(* Logix 5000 AddOnInstructionDefinition export Banner_T30RKU_Param_v4; software revision 33.00 *)

TYPE Banner_IOL_Port_v4 :   // UDT that has all of the data items necessary to communicate with a specific Port on a IO-Link Master
STRUCT
   Port_Controlled : INT;   // Each bit represents a port on an IO-Link Master. Set to 1 to tell AOI to control that port.
   Port_Activate : INT;   // Each bit represents a port on an IO-Link Master. When ON that port will process any commands in queue.
   Port_Read : INT;   // Each bit represents a port on an IO-Link Master. Used to determine when device AOI has requested a Read command.
   Port_Write : INT;   // Each bit represents a port on an IO-Link Master. Used to determine when device AOI has requested a Write command.
   Port_RW_Complete : INT;   // Each bit represents a port on an IO-Link Master. Tells device AOI that Read or Write request has been completed.
   Port_Device_Read : INT;
   Data_Transfer : SINT[190];   // Array to transfer data from IO-Master to device AOIs.
END_STRUCT
END_TYPE

TYPE Banner_T30RKU_RD_v4 :   // UDT that stores the Read Data for a T30RKU.
STRUCT
   Master_Cycle_Time : INT;
   Min_Cycle_Time : INT;
   M_Sequence_Capability : INT;
   IO_Link_Version_ID : INT;
   Process_Data_Input_Length : INT;
   Process_Data_Output_Length : INT;
   Combined_Vendor_ID : DINT;   // IO-Link Vendor ID
   Vendor_ID1 : INT;
   Vendor_ID2 : INT;
   Combined_Device_ID : DINT;   // IO-Link Device ID
   Device_ID1 : INT;
   Device_ID2 : INT;
   Device_ID3 : INT;
   Serial_Number : STRING;
   Teach_State : SINT;
   SP1_TP1 : SINT;
   SP1_TP2 : SINT;
   SP2_TP1 : SINT;
   SP2_TP2 : SINT;
   Distance_Meaurement : DINT;
   Excess_Gain : DINT;   // Amount of singla measured over the minimum threshold.
   Stability : SINT;
   Fault_Status : SINT;   // 0 = No Fault, 1 = Fault Present
   Analog_Output_Value : DINT;
   Temperature : DINT;
   Last_Taught_Temperature : DINT;   // Internal Temperature the last time device was taught.
   All_Time_Run_Time : DINT;   // Read only counter that tracks the total time sensor has been running since manufacture. Value in Hours.
   MDC_Lower_Limit : DINT;
   MDC_Upper_Limit : DINT;
   MDC_Unit : INT;
   MDC_Scale : SINT;
END_STRUCT
END_TYPE

TYPE Banner_T30RKU_v4 :   // All of the parameters for a T30RKU.
STRUCT
   Initial_Global_Read : BOOL;   // Determines if all of the IO-Link data has been read into the PLC yet
   Command : INT;   // Value placed in here will activate a read or write to a specifc IO-Link Index
   Read_Data : Banner_T30RKU_RD_v4;   // Read Only Data
   Write_Data : Banner_T30RKU_WD_v4;   // Write Data
   Archive : Banner_T30RKU_WD_v4;   // Archive Data
   Reset : BOOL;   // Resets AOI. This will force a complete parameter read of the sensor.
END_STRUCT
END_TYPE

TYPE Banner_T30RKU_WD_v4 :   // UDT that stores the Write Data for a T30RKU.
STRUCT
   System_Command : INT;   // See IODD file for list of commands that can be activated via the System Command interface
   Parameter_Access_Lock : SINT;   // Write access to all parameters is prohibited while value is 1. Only this parameter can be adjusted when value is 1.
   Data_Storage_Lock : SINT;   // Automatic data storage is disabled when this value is equal to 1. Read access is not affected.
   Local_Parameterization_Lock : SINT;   // Parameterization via local control elements on device is disabled.
   Local_User_Interface_Lock : SINT;   // Operation of local user interface is disabled.
   Function_Tag : STRING;
   Location_Tag : STRING;
   Teach_in_Channel : SINT;   // 0 = Default, 1 = BDC1, 192 = AO1
   BDC1_Setpoint_1 : DINT;   // 0 to 15000. SP1 switch point in Switch or Window mode.
   BDC1_Setpoint_2 : DINT;   // 0 to 15000. SP2 switch point in Window mode only.
   BDC1_Switchpoint_Logic : INT;   // 0 = Light Operate, 1 = Dark Operate
   BDC1_Mode : SINT;   // 1 = Switch Mode/Single Mode, 2 = Window Mode
   BDC1_Hysteresis : INT;   // 0 to 15000
   Response_Speed : SINT;   // 0 = Fast, 1 = Medium, 2 = Slow
   Peak_Select_Mode : SINT;   // 0 = Strongest Peak, 1 = First Peak
   Sensor_Lockout : SINT;   // 0 = Unlocked, 1 = Locked
   Output_Polarity : SINT;   // 0 = NPN, 1 = PNP
   Process_Data_Filter_Time : INT;
   Process_Data_Layout : SINT;   // 0 = Digital Measurement Sensor, 1 = Distance and Excess Gain, 2 = Distance and Excess Gain with Binary Data
   Remote_Input_Mode : SINT;   // 0 = Disabled, 1 = Teach
   Amplitude_Threshold : DINT;   // 100 to 5000
   Limit_Filter_Enabled : SINT;   // 0 = Disabled, 1 = Enabled. Rate of change filter for the distance measurement.
   Limit_Filter_Hold_Time : DINT;   // 50 to 60000. Hold time for when distance change exceeds configured window.
   Limit_Filter_Positive_Distance : DINT;   // 0 to 1000. Window size for distance changes going away from sensor (set to 0 to disable)
   Limit_Filter_Negative_Distance : DINT;   // 0 to 1000. Window size for distance changes goin towards sensor (set to 0 to disable)
   BDC1_Delay_Timer_1 : DINT;   // 0 to 60000 ms
   BDC1_Delay_Timer_2 : DINT;   // 0 to 60000 ms
   BDC1_Teach_Offset : DINT;   // -15000 to 15000.
   Resettable_Run_Time : DINT;
   AO1_Setpoint_1 : DINT;   // 300 to 15000.
   AO1_Setpoint_2 : DINT;   // 300 to 15000.
   AO1_Output_Type : INT;   // 0 = 4-20 mA, 128 = 0-10V, 129 = .5-4.5V
   AO1_Slope : SINT;   // 0 = Positive, 1 = Negative
   AO1_Loss_of_Signal : SINT;   // 0 = Hold, 1 = Low, 2 = High
   AO1_Average : SINT;   // 0 = 1, 1 = 2, 2= 4, 3 = 8, 4 = 16, 5 = 32, 6 = 64, 7 = 128, 8 = 256, 9 = 512
   All_Time_Run_Time_Event_Time : DINT;
   Resettable_Run_Time_Event_Time : DINT;
   Active_Sensing_Range_Near : DINT;   // 0 to 16000.
   Active_Sensing_Range_Far : DINT;   // 0 to 16000.
END_STRUCT
END_TYPE

ADD_ON_INSTRUCTION Banner_T30RKU_Param_v4   (* revision 4.1, vendor Banner Engineering *)
// AOI to read and write parameter data to an IO-Link T30R Analog.
VAR_IN_OUT
   T30RKU : Banner_T30RKU_v4; {required}
   Port_Data : Banner_IOL_Port_v4; {required}
END_VAR
VAR_INPUT
   Port : DINT; {required}
END_VAR
VAR
   Local_Control : DINT; {access None}
   Global_Read_Command_Value : INT; {access None}
   Global_Write_Command_Value : INT; {access None}
   Command_Being_Processed : BOOL; {access None}
   Update_Archive : BOOL; {access None}
   Index_Write_Inprocess : DINT; {access None}
   Index_Write_Control : DINT; {access None}
   Inprocess_Index : DINT; {access None}
END_VAR

ROUTINE Logic   (* ladder *)
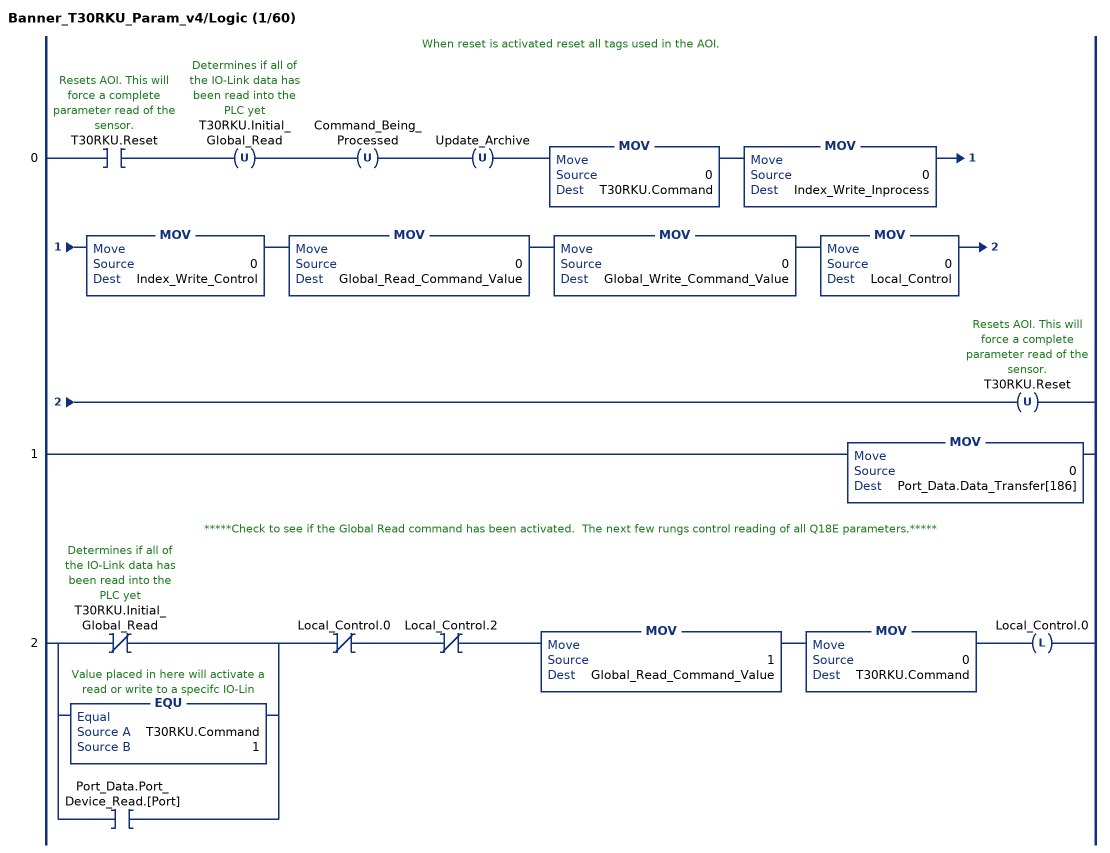
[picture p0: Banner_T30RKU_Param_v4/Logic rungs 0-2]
   // When reset is activated reset all tags used in the AOI.
   0: XIC(T30RKU.Reset)OTU(T30RKU.Initial_Global_Read)OTU(Command_Being_Processed)OTU(Update_Archive)MOV(0,T30RKU.Command)MOV(0,Index_Write_Inprocess)MOV(0,Index_Write_Control)MOV(0,Global_Read_Command_Value)MOV(0,Global_Write_Command_Value)MOV(0,Local_Control)OTU(T30RKU.Reset);
   1: MOV(0,Port_Data.Data_Transfer[186]);
   // *****Check to see if the Global Read command has been activated.  The next few rungs control reading of all Q18E parameters.*****
   2: [XIO(T30RKU.Initial_Global_Read) ,EQU(T30RKU.Command,1) ,XIC(Port_Data.Port_Device_Read.[Port]) ]XIO(Local_Control.0)XIO(Local_Control.2)MOV(1,Global_Read_Command_Value)MOV(0,T30RKU.Command)OTL(Local_Control.0);
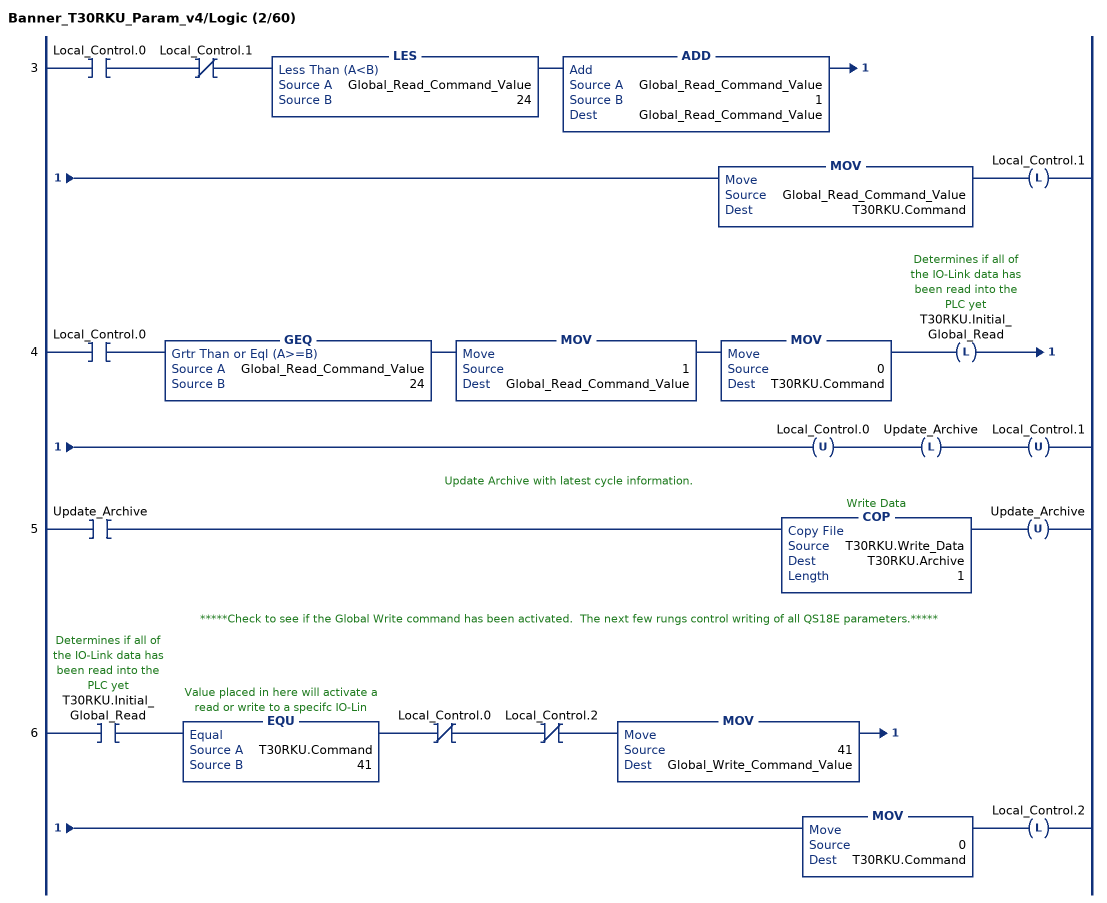
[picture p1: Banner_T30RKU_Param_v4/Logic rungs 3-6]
   3: XIC(Local_Control.0)XIO(Local_Control.1)LES(Global_Read_Command_Value,24)ADD(Global_Read_Command_Value,1,Global_Read_Command_Value)MOV(Global_Read_Command_Value,T30RKU.Command)OTL(Local_Control.1);
   4: XIC(Local_Control.0)GEQ(Global_Read_Command_Value,24)MOV(1,Global_Read_Command_Value)MOV(0,T30RKU.Command)OTL(T30RKU.Initial_Global_Read)OTU(Local_Control.0)OTL(Update_Archive)OTU(Local_Control.1);
   // Update Archive with latest cycle information.
   5: XIC(Update_Archive)COP(T30RKU.Write_Data,T30RKU.Archive,1)OTU(Update_Archive);
   // *****Check to see if the Global Write command has been activated.  The next few rungs control writing of all QS18E parameters.*****
   6: XIC(T30RKU.Initial_Global_Read)EQU(T30RKU.Command,41)XIO(Local_Control.0)XIO(Local_Control.2)MOV(41,Global_Write_Command_Value)MOV(0,T30RKU.Command)OTL(Local_Control.2);
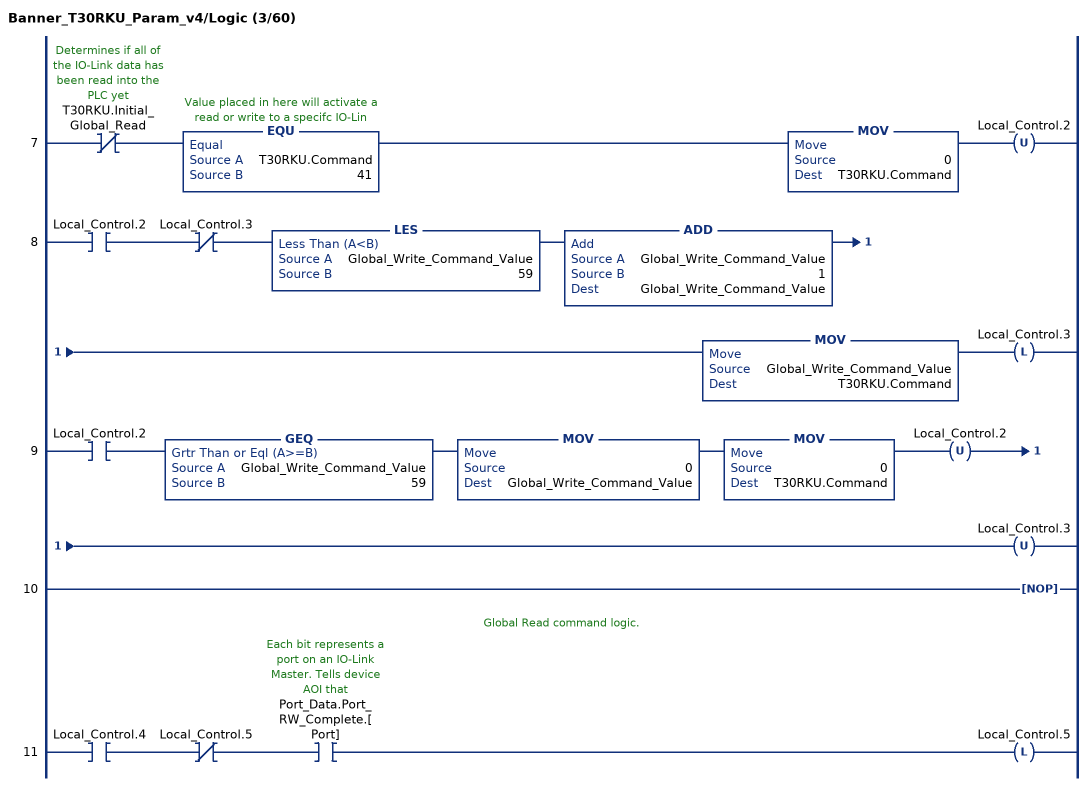
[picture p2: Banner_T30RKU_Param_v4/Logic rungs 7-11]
   7: XIO(T30RKU.Initial_Global_Read)EQU(T30RKU.Command,41)MOV(0,T30RKU.Command)OTU(Local_Control.2);
   8: XIC(Local_Control.2)XIO(Local_Control.3)LES(Global_Write_Command_Value,59)ADD(Global_Write_Command_Value,1,Global_Write_Command_Value)MOV(Global_Write_Command_Value,T30RKU.Command)OTL(Local_Control.3);
   9: XIC(Local_Control.2)GEQ(Global_Write_Command_Value,59)MOV(0,Global_Write_Command_Value)MOV(0,T30RKU.Command)OTU(Local_Control.2)OTU(Local_Control.3);
   10: NOP();
   // Global Read command logic.
   11: XIC(Local_Control.4)XIO(Local_Control.5)XIC(Port_Data.Port_RW_Complete.[Port])OTL(Local_Control.5);
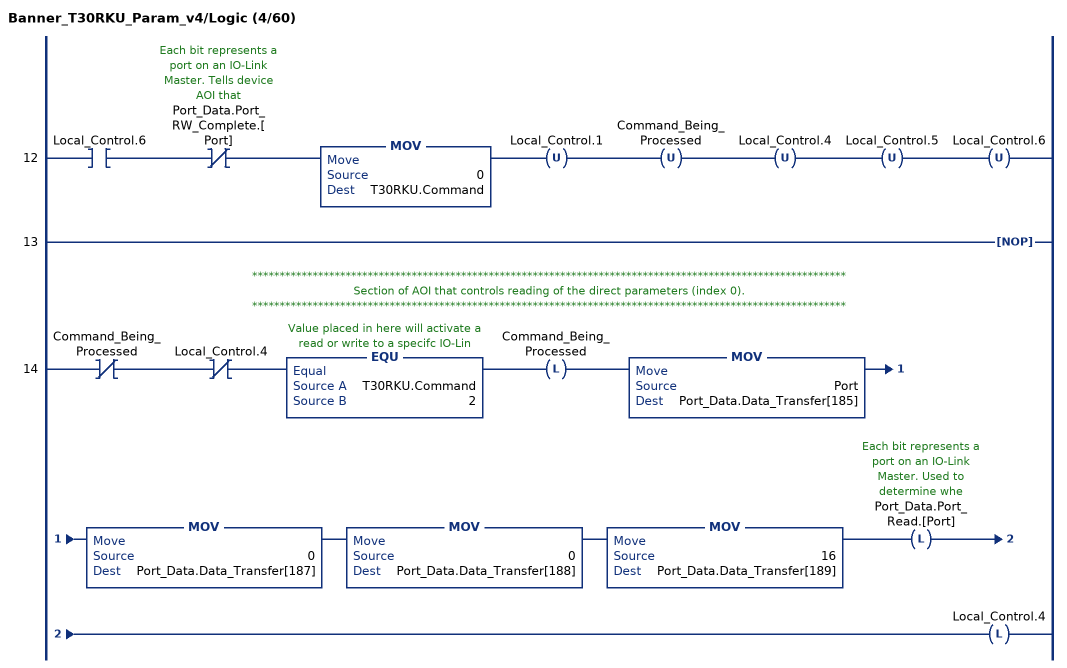
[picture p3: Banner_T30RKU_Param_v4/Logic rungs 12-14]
   12: XIC(Local_Control.6)XIO(Port_Data.Port_RW_Complete.[Port])MOV(0,T30RKU.Command)OTU(Local_Control.1)OTU(Command_Being_Processed)OTU(Local_Control.4)OTU(Local_Control.5)OTU(Local_Control.6);
   13: NOP();
   // ************************************************************************************************************
   // Section of AOI that controls reading of the direct parameters (index 0).
   // ************************************************************************************************************
   14: XIO(Command_Being_Processed)XIO(Local_Control.4)EQU(T30RKU.Command,2)OTL(Command_Being_Processed)MOV(Port,Port_Data.Data_Transfer[185])MOV(0,Port_Data.Data_Transfer[187])MOV(0,Port_Data.Data_Transfer[188])MOV(16,Port_Data.Data_Transfer[189])OTL(Port_Data.Port_Read.[Port])OTL(Local_Control.4);
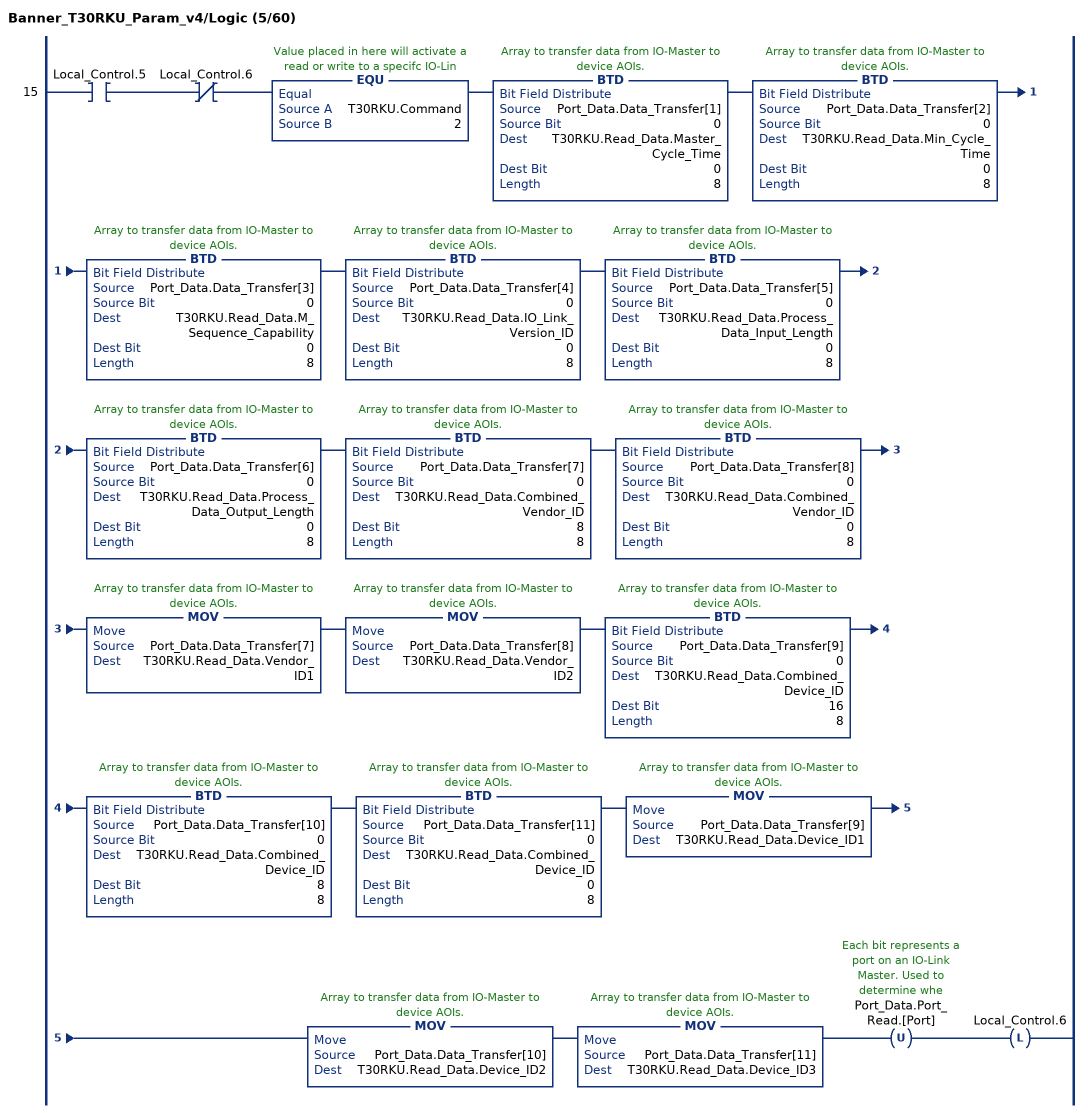
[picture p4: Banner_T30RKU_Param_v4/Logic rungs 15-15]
   15: XIC(Local_Control.5)XIO(Local_Control.6)EQU(T30RKU.Command,2)BTD(Port_Data.Data_Transfer[1],0,T30RKU.Read_Data.Master_Cycle_Time,0,8)BTD(Port_Data.Data_Transfer[2],0,T30RKU.Read_Data.Min_Cycle_Time,0,8)BTD(Port_Data.Data_Transfer[3],0,T30RKU.Read_Data.M_Sequence_Capability,0,8)BTD(Port_Data.Data_Transfer[4],0,T30RKU.Read_Data.IO_Link_Version_ID,0,8)BTD(Port_Data.Data_Transfer[5],0,T30RKU.Read_Data.Process_Data_Input_Length,0,8)BTD(Port_Data.Data_Transfer[6],0,T30RKU.Read_Data.Process_Data_Output_Length,0,8)BTD(Port_Data.Data_Transfer[7],0,T30RKU.Read_Data.Combined_Vendor_ID,8,8)BTD(Port_Data.Data_Transfer[8],0,T30RKU.Read_Data.Combined_Vendor_ID,0,8)MOV(Port_Data.Data_Transfer[7],T30RKU.Read_Data.Vendor_ID1)MOV(Port_Data.Data_Transfer[8],T30RKU.Read_Data.Vendor_ID2)BTD(Port_Data.Data_Transfer[9],0,T30RKU.Read_Data.Combined_Device_ID,16,8)BTD(Port_Data.Data_Transfer[10],0,T30RKU.Read_Data.Combined_Device_ID,8,8)BTD(Port_Data.Data_Transfer[11],0,T30RKU.Read_Data.Combined_Device_ID,0,8)MOV(Port_Data.Data_Transfer[9],T30RKU.Read_Data.Device_ID1)MOV(Port_Data.Data_Transfer[10],T30RKU.Read_Data.Device_ID2)MOV(Port_Data.Data_Transfer[11],T30RKU.Read_Data.Device_ID3)OTU(Port_Data.Port_Read.[Port])OTL(Local_Control.6);
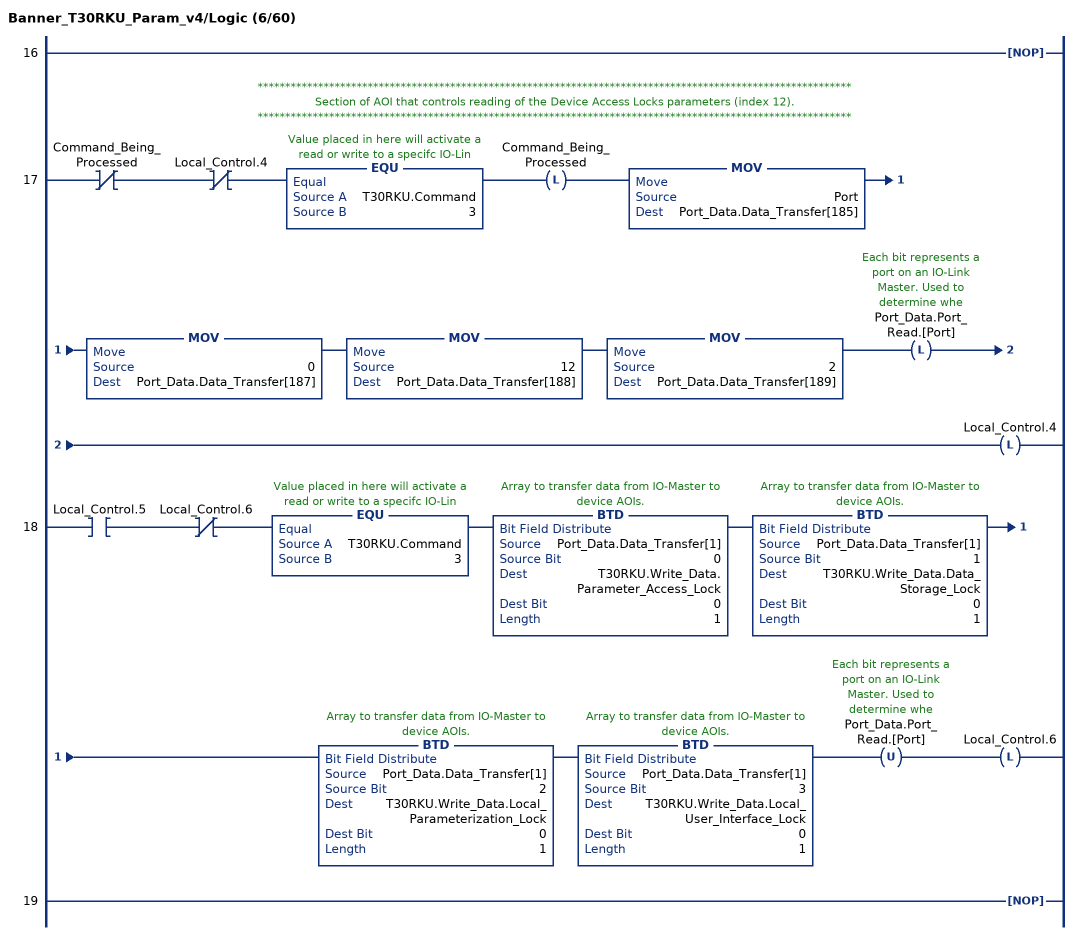
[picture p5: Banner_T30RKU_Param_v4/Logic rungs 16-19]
   16: NOP();
   // ************************************************************************************************************
   // Section of AOI that controls reading of the Device Access Locks parameters (index 12).
   // ************************************************************************************************************
   17: XIO(Command_Being_Processed)XIO(Local_Control.4)EQU(T30RKU.Command,3)OTL(Command_Being_Processed)MOV(Port,Port_Data.Data_Transfer[185])MOV(0,Port_Data.Data_Transfer[187])MOV(12,Port_Data.Data_Transfer[188])MOV(2,Port_Data.Data_Transfer[189])OTL(Port_Data.Port_Read.[Port])OTL(Local_Control.4);
   18: XIC(Local_Control.5)XIO(Local_Control.6)EQU(T30RKU.Command,3)BTD(Port_Data.Data_Transfer[1],0,T30RKU.Write_Data.Parameter_Access_Lock,0,1)BTD(Port_Data.Data_Transfer[1],1,T30RKU.Write_Data.Data_Storage_Lock,0,1)BTD(Port_Data.Data_Transfer[1],2,T30RKU.Write_Data.Local_Parameterization_Lock,0,1)BTD(Port_Data.Data_Transfer[1],3,T30RKU.Write_Data.Local_User_Interface_Lock,0,1)OTU(Port_Data.Port_Read.[Port])OTL(Local_Control.6);
   19: NOP();
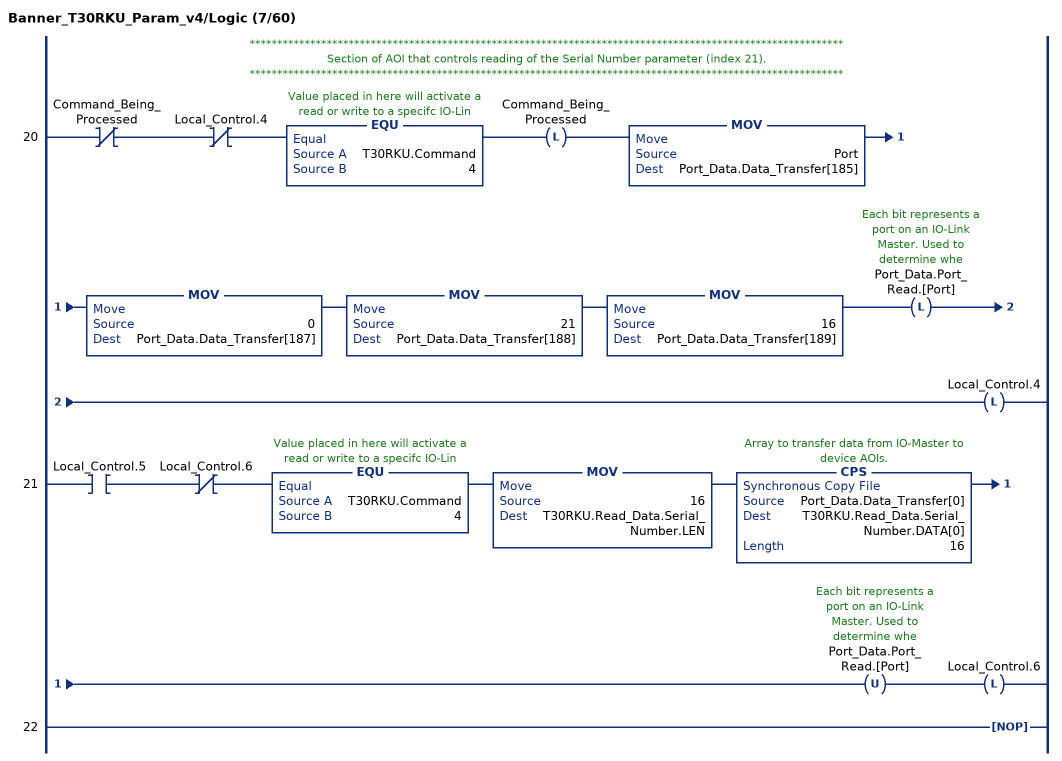
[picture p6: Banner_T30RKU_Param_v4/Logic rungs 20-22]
   // ************************************************************************************************************
   // Section of AOI that controls reading of the Serial Number parameter (index 21).
   // ************************************************************************************************************
   20: XIO(Command_Being_Processed)XIO(Local_Control.4)EQU(T30RKU.Command,4)OTL(Command_Being_Processed)MOV(Port,Port_Data.Data_Transfer[185])MOV(0,Port_Data.Data_Transfer[187])MOV(21,Port_Data.Data_Transfer[188])MOV(16,Port_Data.Data_Transfer[189])OTL(Port_Data.Port_Read.[Port])OTL(Local_Control.4);
   21: XIC(Local_Control.5)XIO(Local_Control.6)EQU(T30RKU.Command,4)MOV(16,T30RKU.Read_Data.Serial_Number.LEN)CPS(Port_Data.Data_Transfer[0],T30RKU.Read_Data.Serial_Number.DATA[0],16)OTU(Port_Data.Port_Read.[Port])OTL(Local_Control.6);
   22: NOP();
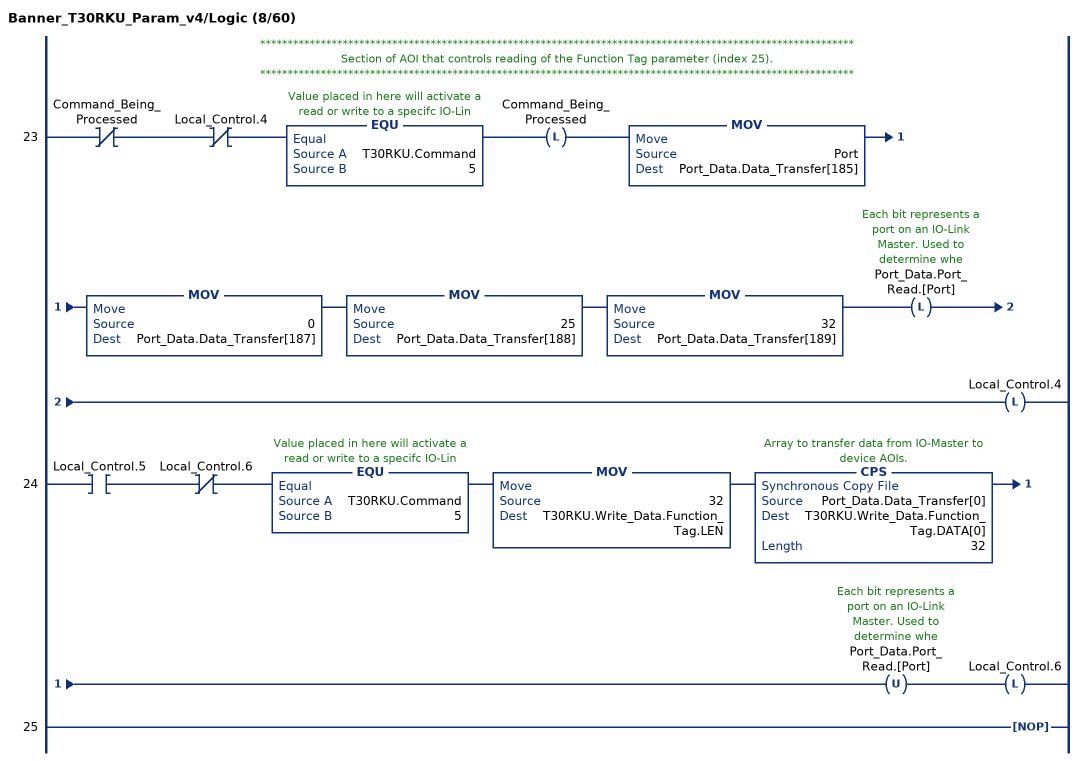
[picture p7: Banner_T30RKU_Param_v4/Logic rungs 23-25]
   // ************************************************************************************************************
   // Section of AOI that controls reading of the Function Tag parameter (index 25).
   // ************************************************************************************************************
   23: XIO(Command_Being_Processed)XIO(Local_Control.4)EQU(T30RKU.Command,5)OTL(Command_Being_Processed)MOV(Port,Port_Data.Data_Transfer[185])MOV(0,Port_Data.Data_Transfer[187])MOV(25,Port_Data.Data_Transfer[188])MOV(32,Port_Data.Data_Transfer[189])OTL(Port_Data.Port_Read.[Port])OTL(Local_Control.4);
   24: XIC(Local_Control.5)XIO(Local_Control.6)EQU(T30RKU.Command,5)MOV(32,T30RKU.Write_Data.Function_Tag.LEN)CPS(Port_Data.Data_Transfer[0],T30RKU.Write_Data.Function_Tag.DATA[0],32)OTU(Port_Data.Port_Read.[Port])OTL(Local_Control.6);
   25: NOP();
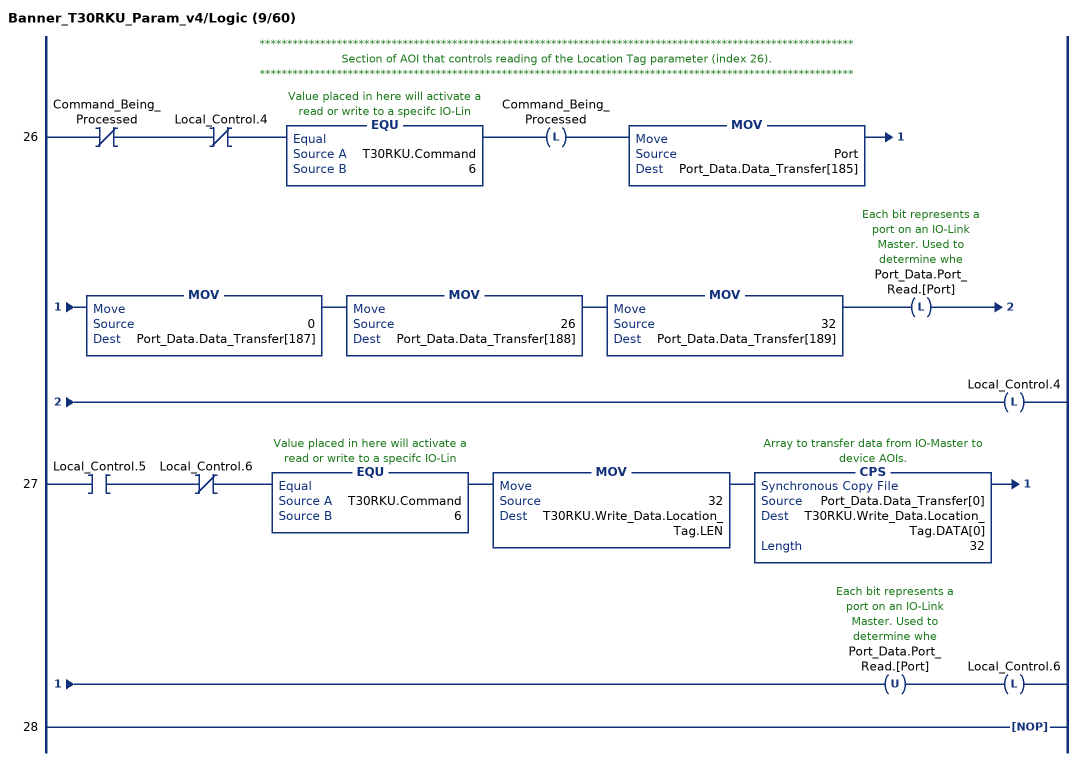
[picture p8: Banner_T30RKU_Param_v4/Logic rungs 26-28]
   // ************************************************************************************************************
   // Section of AOI that controls reading of the Location Tag parameter (index 26).
   // ************************************************************************************************************
   26: XIO(Command_Being_Processed)XIO(Local_Control.4)EQU(T30RKU.Command,6)OTL(Command_Being_Processed)MOV(Port,Port_Data.Data_Transfer[185])MOV(0,Port_Data.Data_Transfer[187])MOV(26,Port_Data.Data_Transfer[188])MOV(32,Port_Data.Data_Transfer[189])OTL(Port_Data.Port_Read.[Port])OTL(Local_Control.4);
   27: XIC(Local_Control.5)XIO(Local_Control.6)EQU(T30RKU.Command,6)MOV(32,T30RKU.Write_Data.Location_Tag.LEN)CPS(Port_Data.Data_Transfer[0],T30RKU.Write_Data.Location_Tag.DATA[0],32)OTU(Port_Data.Port_Read.[Port])OTL(Local_Control.6);
   28: NOP();
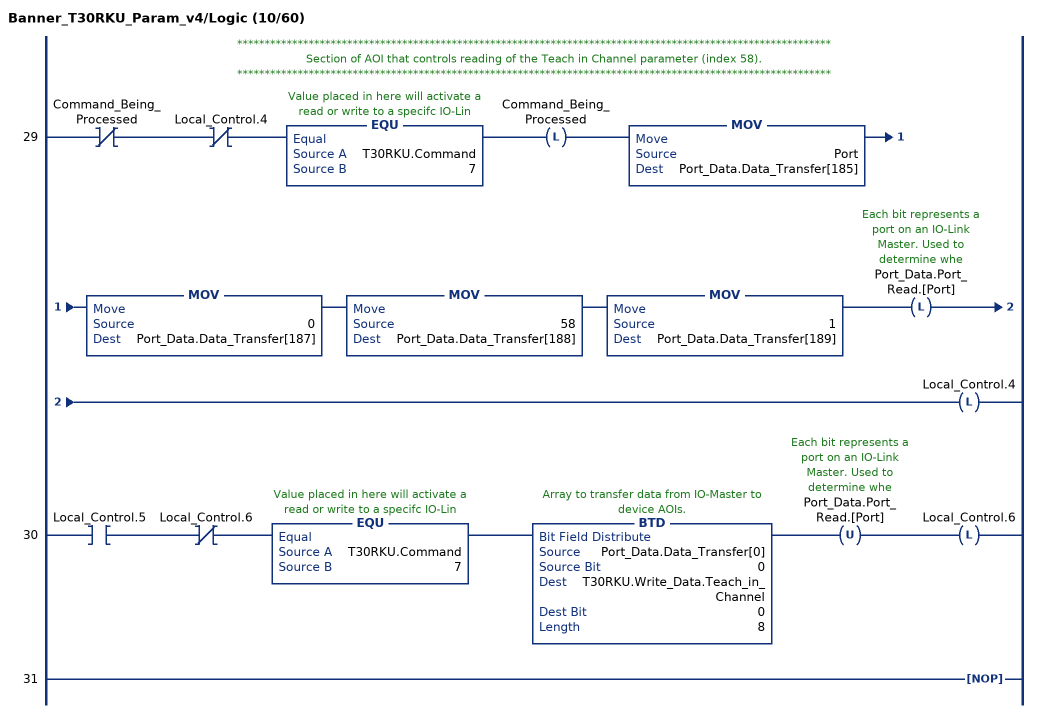
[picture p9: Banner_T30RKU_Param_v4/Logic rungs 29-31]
   // ************************************************************************************************************
   // Section of AOI that controls reading of the Teach in Channel parameter (index 58).
   // ************************************************************************************************************
   29: XIO(Command_Being_Processed)XIO(Local_Control.4)EQU(T30RKU.Command,7)OTL(Command_Being_Processed)MOV(Port,Port_Data.Data_Transfer[185])MOV(0,Port_Data.Data_Transfer[187])MOV(58,Port_Data.Data_Transfer[188])MOV(1,Port_Data.Data_Transfer[189])OTL(Port_Data.Port_Read.[Port])OTL(Local_Control.4);
   30: XIC(Local_Control.5)XIO(Local_Control.6)EQU(T30RKU.Command,7)BTD(Port_Data.Data_Transfer[0],0,T30RKU.Write_Data.Teach_in_Channel,0,8)OTU(Port_Data.Port_Read.[Port])OTL(Local_Control.6);
   31: NOP();
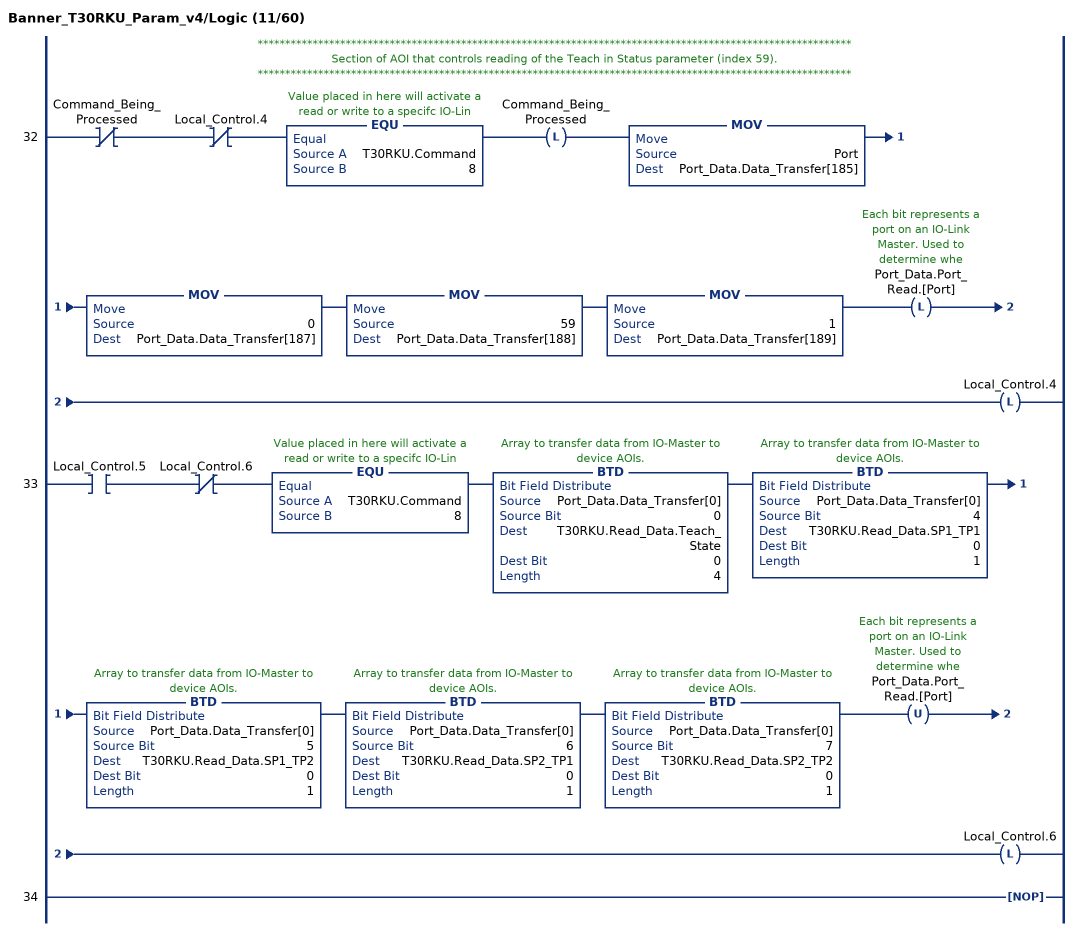
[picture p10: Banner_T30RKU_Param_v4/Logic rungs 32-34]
   // ************************************************************************************************************
   // Section of AOI that controls reading of the Teach in Status parameter (index 59).
   // ************************************************************************************************************
   32: XIO(Command_Being_Processed)XIO(Local_Control.4)EQU(T30RKU.Command,8)OTL(Command_Being_Processed)MOV(Port,Port_Data.Data_Transfer[185])MOV(0,Port_Data.Data_Transfer[187])MOV(59,Port_Data.Data_Transfer[188])MOV(1,Port_Data.Data_Transfer[189])OTL(Port_Data.Port_Read.[Port])OTL(Local_Control.4);
   33: XIC(Local_Control.5)XIO(Local_Control.6)EQU(T30RKU.Command,8)BTD(Port_Data.Data_Transfer[0],0,T30RKU.Read_Data.Teach_State,0,4)BTD(Port_Data.Data_Transfer[0],4,T30RKU.Read_Data.SP1_TP1,0,1)BTD(Port_Data.Data_Transfer[0],5,T30RKU.Read_Data.SP1_TP2,0,1)BTD(Port_Data.Data_Transfer[0],6,T30RKU.Read_Data.SP2_TP1,0,1)BTD(Port_Data.Data_Transfer[0],7,T30RKU.Read_Data.SP2_TP2,0,1)OTU(Port_Data.Port_Read.[Port])OTL(Local_Control.6);
   34: NOP();
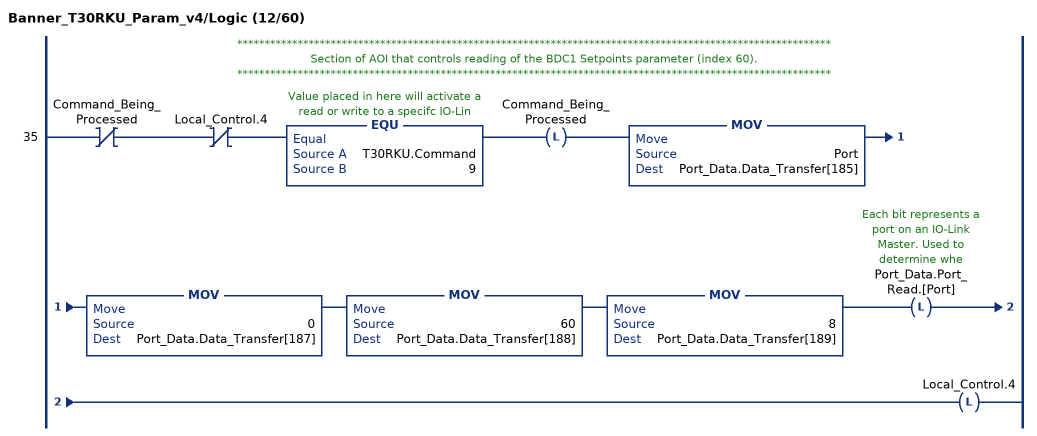
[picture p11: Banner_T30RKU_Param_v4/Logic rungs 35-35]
   // ************************************************************************************************************
   // Section of AOI that controls reading of the BDC1 Setpoints parameter (index 60).
   // ************************************************************************************************************
   35: XIO(Command_Being_Processed)XIO(Local_Control.4)EQU(T30RKU.Command,9)OTL(Command_Being_Processed)MOV(Port,Port_Data.Data_Transfer[185])MOV(0,Port_Data.Data_Transfer[187])MOV(60,Port_Data.Data_Transfer[188])MOV(8,Port_Data.Data_Transfer[189])OTL(Port_Data.Port_Read.[Port])OTL(Local_Control.4);
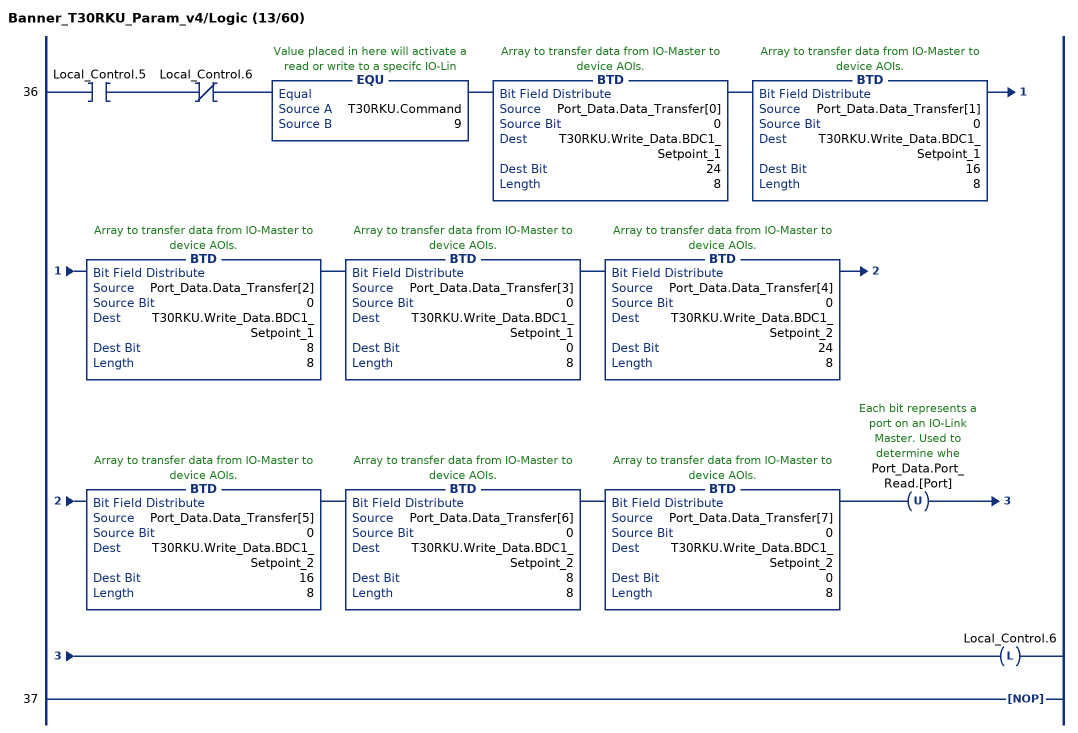
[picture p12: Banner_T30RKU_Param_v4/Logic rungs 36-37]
   36: XIC(Local_Control.5)XIO(Local_Control.6)EQU(T30RKU.Command,9)BTD(Port_Data.Data_Transfer[0],0,T30RKU.Write_Data.BDC1_Setpoint_1,24,8)BTD(Port_Data.Data_Transfer[1],0,T30RKU.Write_Data.BDC1_Setpoint_1,16,8)BTD(Port_Data.Data_Transfer[2],0,T30RKU.Write_Data.BDC1_Setpoint_1,8,8)BTD(Port_Data.Data_Transfer[3],0,T30RKU.Write_Data.BDC1_Setpoint_1,0,8)BTD(Port_Data.Data_Transfer[4],0,T30RKU.Write_Data.BDC1_Setpoint_2,24,8)BTD(Port_Data.Data_Transfer[5],0,T30RKU.Write_Data.BDC1_Setpoint_2,16,8)BTD(Port_Data.Data_Transfer[6],0,T30RKU.Write_Data.BDC1_Setpoint_2,8,8)BTD(Port_Data.Data_Transfer[7],0,T30RKU.Write_Data.BDC1_Setpoint_2,0,8)OTU(Port_Data.Port_Read.[Port])OTL(Local_Control.6);
   37: NOP();
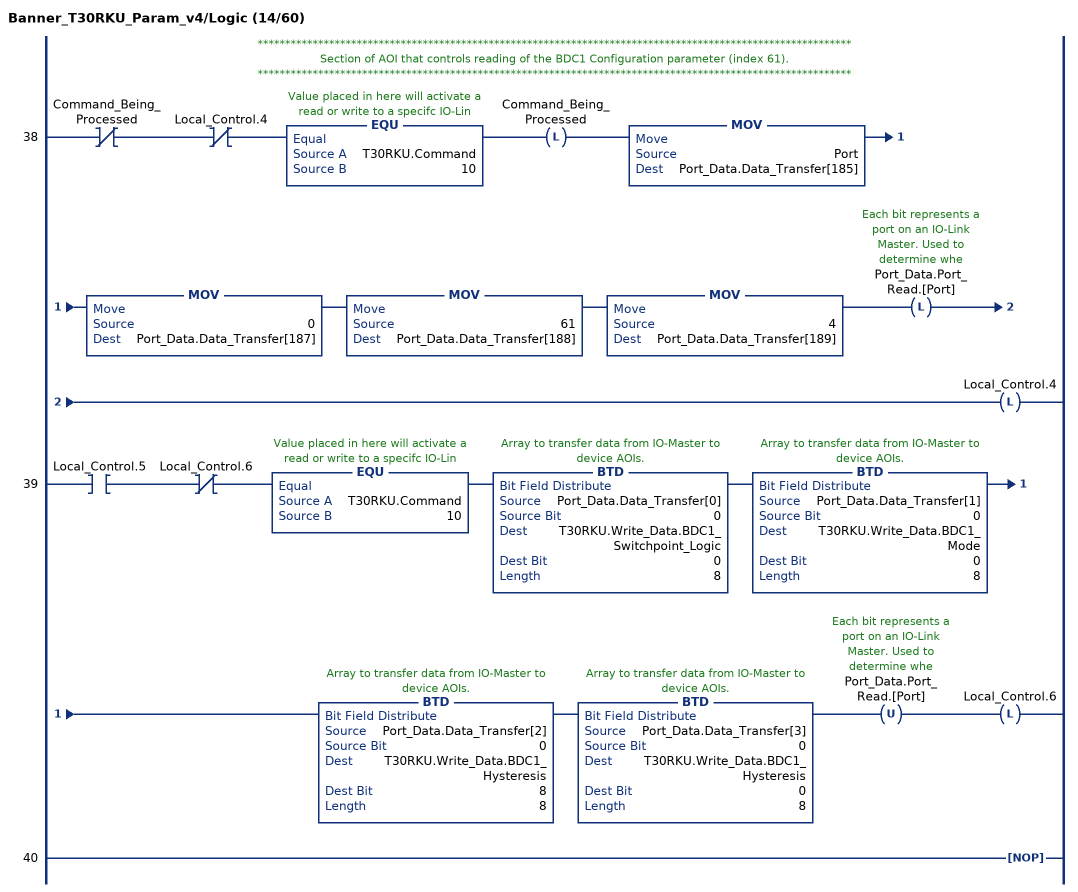
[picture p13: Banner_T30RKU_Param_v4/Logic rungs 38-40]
   // ************************************************************************************************************
   // Section of AOI that controls reading of the BDC1 Configuration parameter (index 61).
   // ************************************************************************************************************
   38: XIO(Command_Being_Processed)XIO(Local_Control.4)EQU(T30RKU.Command,10)OTL(Command_Being_Processed)MOV(Port,Port_Data.Data_Transfer[185])MOV(0,Port_Data.Data_Transfer[187])MOV(61,Port_Data.Data_Transfer[188])MOV(4,Port_Data.Data_Transfer[189])OTL(Port_Data.Port_Read.[Port])OTL(Local_Control.4);
   39: XIC(Local_Control.5)XIO(Local_Control.6)EQU(T30RKU.Command,10)BTD(Port_Data.Data_Transfer[0],0,T30RKU.Write_Data.BDC1_Switchpoint_Logic,0,8)BTD(Port_Data.Data_Transfer[1],0,T30RKU.Write_Data.BDC1_Mode,0,8)BTD(Port_Data.Data_Transfer[2],0,T30RKU.Write_Data.BDC1_Hysteresis,8,8)BTD(Port_Data.Data_Transfer[3],0,T30RKU.Write_Data.BDC1_Hysteresis,0,8)OTU(Port_Data.Port_Read.[Port])OTL(Local_Control.6);
   40: NOP();
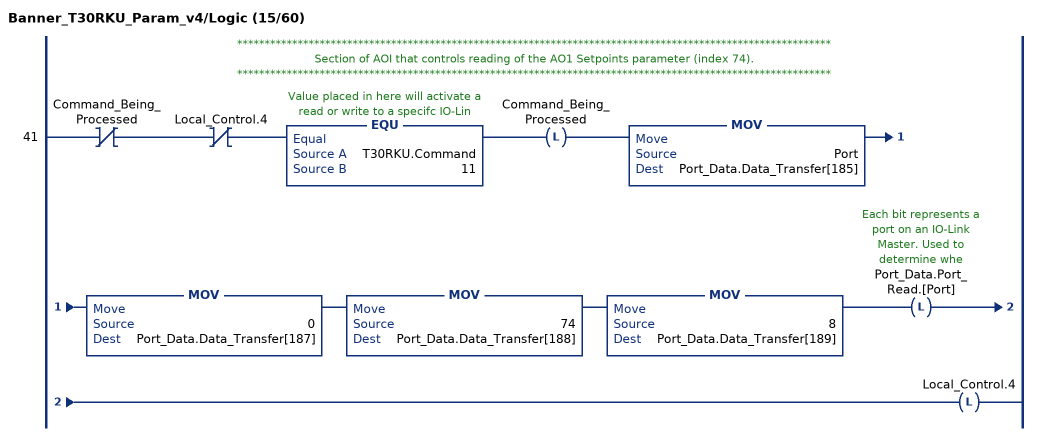
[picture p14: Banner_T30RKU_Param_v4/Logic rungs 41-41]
   // ************************************************************************************************************
   // Section of AOI that controls reading of the AO1 Setpoints parameter (index 74).
   // ************************************************************************************************************
   41: XIO(Command_Being_Processed)XIO(Local_Control.4)EQU(T30RKU.Command,11)OTL(Command_Being_Processed)MOV(Port,Port_Data.Data_Transfer[185])MOV(0,Port_Data.Data_Transfer[187])MOV(74,Port_Data.Data_Transfer[188])MOV(8,Port_Data.Data_Transfer[189])OTL(Port_Data.Port_Read.[Port])OTL(Local_Control.4);
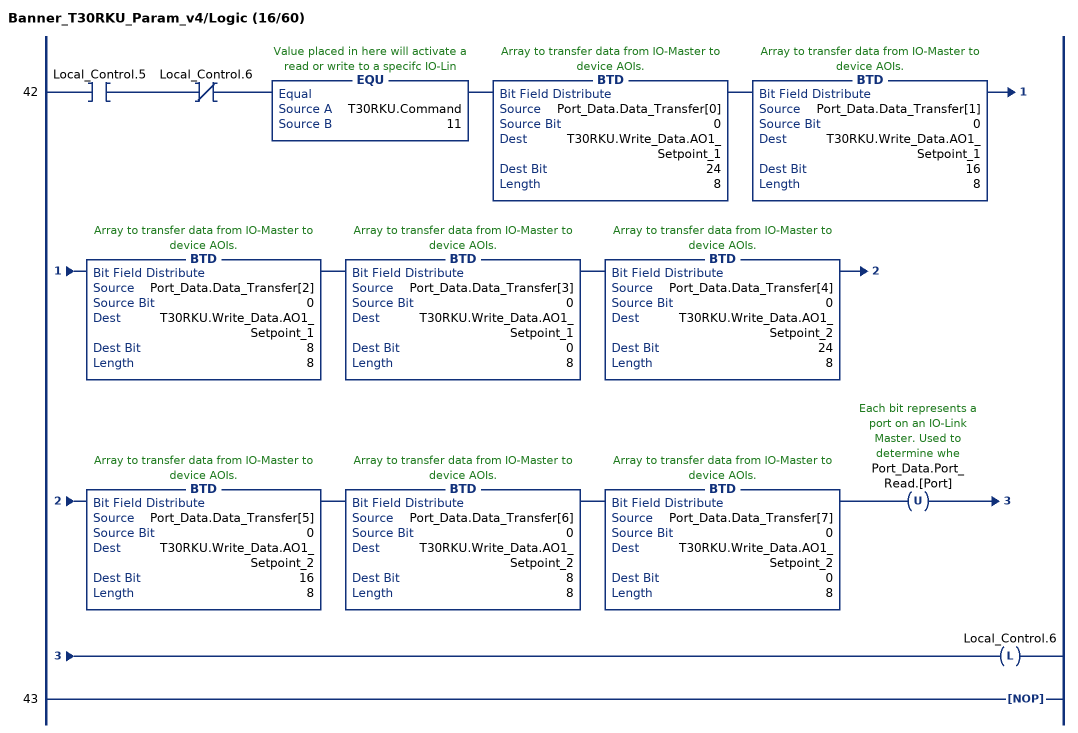
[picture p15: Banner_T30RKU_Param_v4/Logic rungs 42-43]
   42: XIC(Local_Control.5)XIO(Local_Control.6)EQU(T30RKU.Command,11)BTD(Port_Data.Data_Transfer[0],0,T30RKU.Write_Data.AO1_Setpoint_1,24,8)BTD(Port_Data.Data_Transfer[1],0,T30RKU.Write_Data.AO1_Setpoint_1,16,8)BTD(Port_Data.Data_Transfer[2],0,T30RKU.Write_Data.AO1_Setpoint_1,8,8)BTD(Port_Data.Data_Transfer[3],0,T30RKU.Write_Data.AO1_Setpoint_1,0,8)BTD(Port_Data.Data_Transfer[4],0,T30RKU.Write_Data.AO1_Setpoint_2,24,8)BTD(Port_Data.Data_Transfer[5],0,T30RKU.Write_Data.AO1_Setpoint_2,16,8)BTD(Port_Data.Data_Transfer[6],0,T30RKU.Write_Data.AO1_Setpoint_2,8,8)BTD(Port_Data.Data_Transfer[7],0,T30RKU.Write_Data.AO1_Setpoint_2,0,8)OTU(Port_Data.Port_Read.[Port])OTL(Local_Control.6);
   43: NOP();
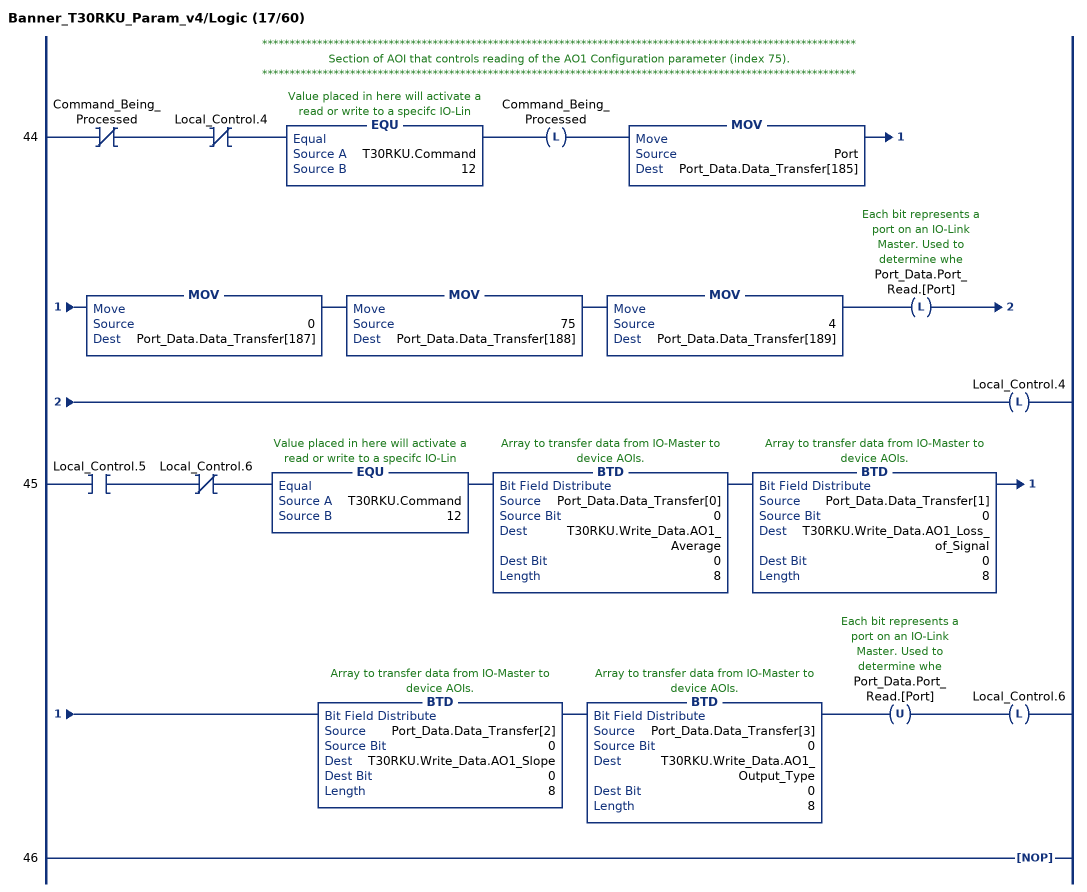
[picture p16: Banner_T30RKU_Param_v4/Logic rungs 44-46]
   // ************************************************************************************************************
   // Section of AOI that controls reading of the AO1 Configuration parameter (index 75).
   // ************************************************************************************************************
   44: XIO(Command_Being_Processed)XIO(Local_Control.4)EQU(T30RKU.Command,12)OTL(Command_Being_Processed)MOV(Port,Port_Data.Data_Transfer[185])MOV(0,Port_Data.Data_Transfer[187])MOV(75,Port_Data.Data_Transfer[188])MOV(4,Port_Data.Data_Transfer[189])OTL(Port_Data.Port_Read.[Port])OTL(Local_Control.4);
   45: XIC(Local_Control.5)XIO(Local_Control.6)EQU(T30RKU.Command,12)BTD(Port_Data.Data_Transfer[0],0,T30RKU.Write_Data.AO1_Average,0,8)BTD(Port_Data.Data_Transfer[1],0,T30RKU.Write_Data.AO1_Loss_of_Signal,0,8)BTD(Port_Data.Data_Transfer[2],0,T30RKU.Write_Data.AO1_Slope,0,8)BTD(Port_Data.Data_Transfer[3],0,T30RKU.Write_Data.AO1_Output_Type,0,8)OTU(Port_Data.Port_Read.[Port])OTL(Local_Control.6);
   46: NOP();
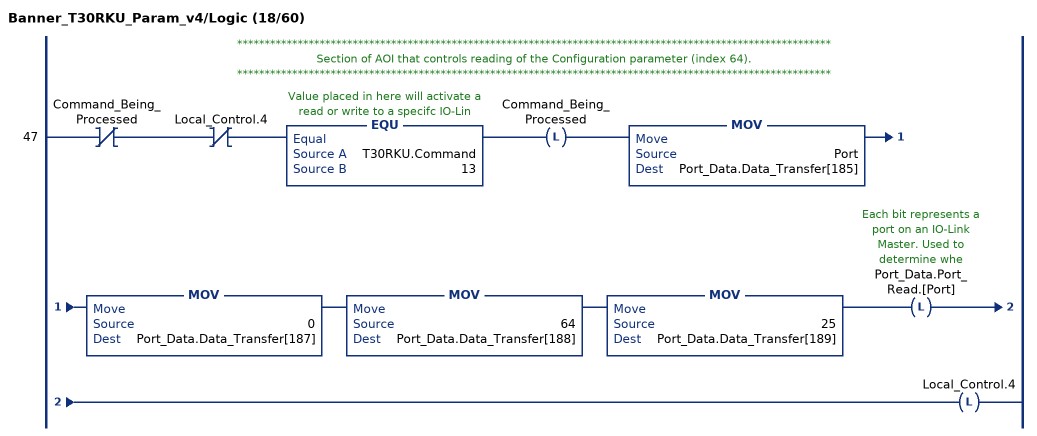
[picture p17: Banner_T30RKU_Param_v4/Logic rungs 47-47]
   // ************************************************************************************************************
   // Section of AOI that controls reading of the Configuration parameter (index 64).
   // ************************************************************************************************************
   47: XIO(Command_Being_Processed)XIO(Local_Control.4)EQU(T30RKU.Command,13)OTL(Command_Being_Processed)MOV(Port,Port_Data.Data_Transfer[185])MOV(0,Port_Data.Data_Transfer[187])MOV(64,Port_Data.Data_Transfer[188])MOV(25,Port_Data.Data_Transfer[189])OTL(Port_Data.Port_Read.[Port])OTL(Local_Control.4);
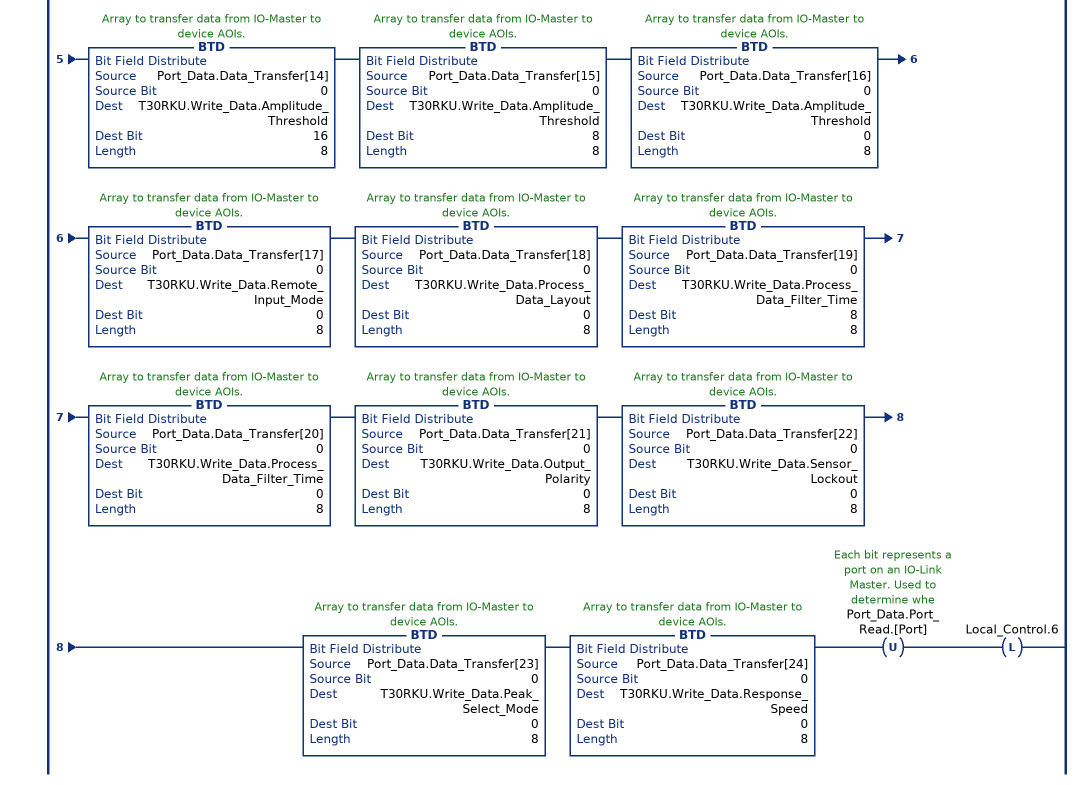
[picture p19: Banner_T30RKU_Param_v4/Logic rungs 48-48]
   48: XIC(Local_Control.5)XIO(Local_Control.6)EQU(T30RKU.Command,13)BTD(Port_Data.Data_Transfer[0],0,T30RKU.Write_Data.Limit_Filter_Negative_Distance,24,8)BTD(Port_Data.Data_Transfer[1],0,T30RKU.Write_Data.Limit_Filter_Negative_Distance,16,8)BTD(Port_Data.Data_Transfer[2],0,T30RKU.Write_Data.Limit_Filter_Negative_Distance,8,8)BTD(Port_Data.Data_Transfer[3],0,T30RKU.Write_Data.Limit_Filter_Negative_Distance,0,8)BTD(Port_Data.Data_Transfer[4],0,T30RKU.Write_Data.Limit_Filter_Positive_Distance,24,8)BTD(Port_Data.Data_Transfer[5],0,T30RKU.Write_Data.Limit_Filter_Positive_Distance,16,8)BTD(Port_Data.Data_Transfer[6],0,T30RKU.Write_Data.Limit_Filter_Positive_Distance,8,8)BTD(Port_Data.Data_Transfer[7],0,T30RKU.Write_Data.Limit_Filter_Positive_Distance,0,8)BTD(Port_Data.Data_Transfer[8],0,T30RKU.Write_Data.Limit_Filter_Hold_Time,24,8)BTD(Port_Data.Data_Transfer[9],0,T30RKU.Write_Data.Limit_Filter_Hold_Time,16,8)BTD(Port_Data.Data_Transfer[10],0,T30RKU.Write_Data.Limit_Filter_Hold_Time,8,8)BTD(Port_Data.Data_Transfer[11],0,T30RKU.Write_Data.Limit_Filter_Hold_Time,0,8)BTD(Port_Data.Data_Transfer[12],0,T30RKU.Write_Data.Limit_Filter_Enabled,0,8)BTD(Port_Data.Data_Transfer[13],0,T30RKU.Write_Data.Amplitude_Threshold,24,8)BTD(Port_Data.Data_Transfer[14],0,T30RKU.Write_Data.Amplitude_Threshold,16,8)BTD(Port_Data.Data_Transfer[15],0,T30RKU.Write_Data.Amplitude_Threshold,8,8)BTD(Port_Data.Data_Transfer[16],0,T30RKU.Write_Data.Amplitude_Threshold,0,8)BTD(Port_Data.Data_Transfer[17],0,T30RKU.Write_Data.Remote_Input_Mode,0,8)BTD(Port_Data.Data_Transfer[18],0,T30RKU.Write_Data.Process_Data_Layout,0,8)BTD(Port_Data.Data_Transfer[19],0,T30RKU.Write_Data.Process_Data_Filter_Time,8,8)BTD(Port_Data.Data_Transfer[20],0,T30RKU.Write_Data.Process_Data_Filter_Time,0,8)BTD(Port_Data.Data_Transfer[21],0,T30RKU.Write_Data.Output_Polarity,0,8)BTD(Port_Data.Data_Transfer[22],0,T30RKU.Write_Data.Sensor_Lockout,0,8)BTD(Port_Data.Data_Transfer[23],0,T30RKU.Write_Data.Peak_Select_Mode,0,8)BTD(Port_Data.Data_Transfer[24],0,T30RKU.Write_Data.Response_Speed,0,8)OTU(Port_Data.Port_Read.[Port])OTL(Local_Control.6);
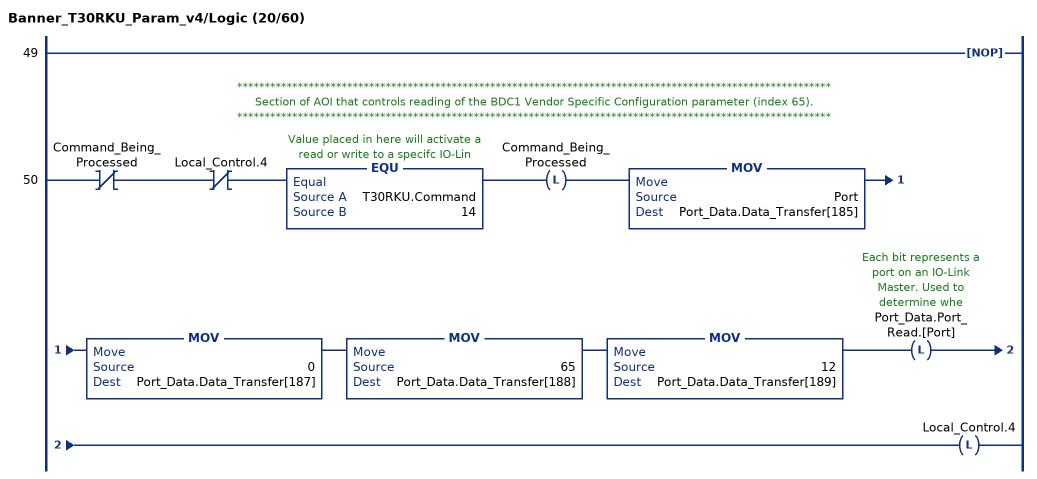
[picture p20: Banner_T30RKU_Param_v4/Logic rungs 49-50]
   49: NOP();
   // ************************************************************************************************************
   // Section of AOI that controls reading of the BDC1 Vendor Specific Configuration parameter (index 65).
   // ************************************************************************************************************
   50: XIO(Command_Being_Processed)XIO(Local_Control.4)EQU(T30RKU.Command,14)OTL(Command_Being_Processed)MOV(Port,Port_Data.Data_Transfer[185])MOV(0,Port_Data.Data_Transfer[187])MOV(65,Port_Data.Data_Transfer[188])MOV(12,Port_Data.Data_Transfer[189])OTL(Port_Data.Port_Read.[Port])OTL(Local_Control.4);
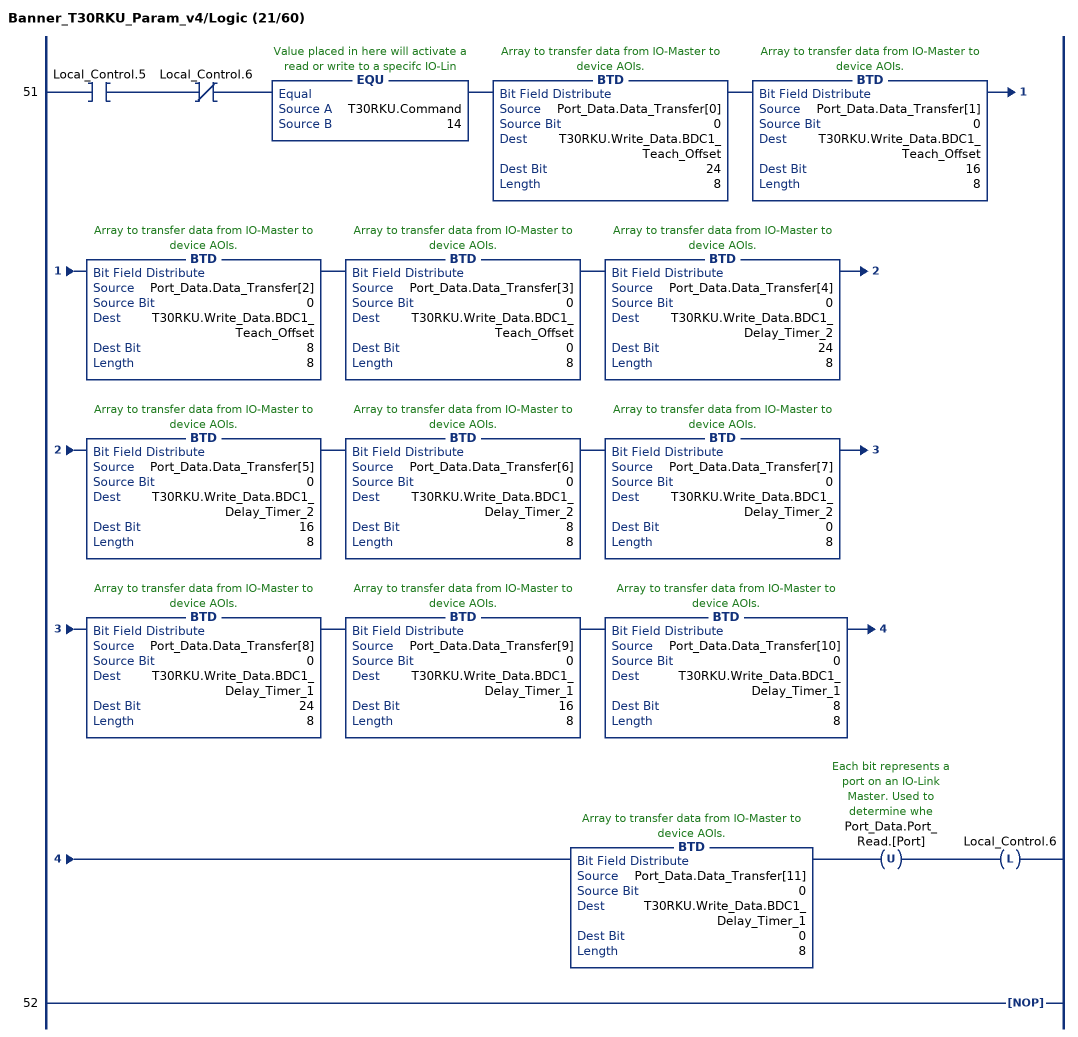
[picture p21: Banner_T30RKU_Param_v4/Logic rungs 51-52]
   51: XIC(Local_Control.5)XIO(Local_Control.6)EQU(T30RKU.Command,14)BTD(Port_Data.Data_Transfer[0],0,T30RKU.Write_Data.BDC1_Teach_Offset,24,8)BTD(Port_Data.Data_Transfer[1],0,T30RKU.Write_Data.BDC1_Teach_Offset,16,8)BTD(Port_Data.Data_Transfer[2],0,T30RKU.Write_Data.BDC1_Teach_Offset,8,8)BTD(Port_Data.Data_Transfer[3],0,T30RKU.Write_Data.BDC1_Teach_Offset,0,8)BTD(Port_Data.Data_Transfer[4],0,T30RKU.Write_Data.BDC1_Delay_Timer_2,24,8)BTD(Port_Data.Data_Transfer[5],0,T30RKU.Write_Data.BDC1_Delay_Timer_2,16,8)BTD(Port_Data.Data_Transfer[6],0,T30RKU.Write_Data.BDC1_Delay_Timer_2,8,8)BTD(Port_Data.Data_Transfer[7],0,T30RKU.Write_Data.BDC1_Delay_Timer_2,0,8)BTD(Port_Data.Data_Transfer[8],0,T30RKU.Write_Data.BDC1_Delay_Timer_1,24,8)BTD(Port_Data.Data_Transfer[9],0,T30RKU.Write_Data.BDC1_Delay_Timer_1,16,8)BTD(Port_Data.Data_Transfer[10],0,T30RKU.Write_Data.BDC1_Delay_Timer_1,8,8)BTD(Port_Data.Data_Transfer[11],0,T30RKU.Write_Data.BDC1_Delay_Timer_1,0,8)OTU(Port_Data.Port_Read.[Port])OTL(Local_Control.6);
   52: NOP();
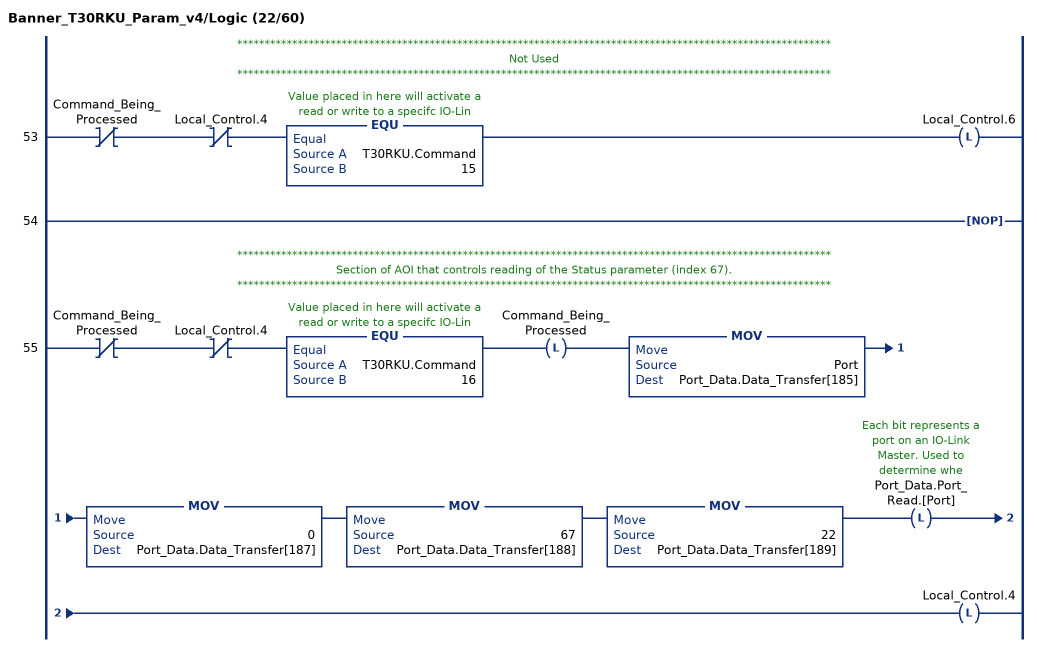
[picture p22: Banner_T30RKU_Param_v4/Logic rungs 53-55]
   // ************************************************************************************************************
   // Not Used
   // ************************************************************************************************************
   53: XIO(Command_Being_Processed)XIO(Local_Control.4)EQU(T30RKU.Command,15)OTL(Local_Control.6);
   54: NOP();
   // ************************************************************************************************************
   // Section of AOI that controls reading of the Status parameter (index 67).
   // ************************************************************************************************************
   55: XIO(Command_Being_Processed)XIO(Local_Control.4)EQU(T30RKU.Command,16)OTL(Command_Being_Processed)MOV(Port,Port_Data.Data_Transfer[185])MOV(0,Port_Data.Data_Transfer[187])MOV(67,Port_Data.Data_Transfer[188])MOV(22,Port_Data.Data_Transfer[189])OTL(Port_Data.Port_Read.[Port])OTL(Local_Control.4);
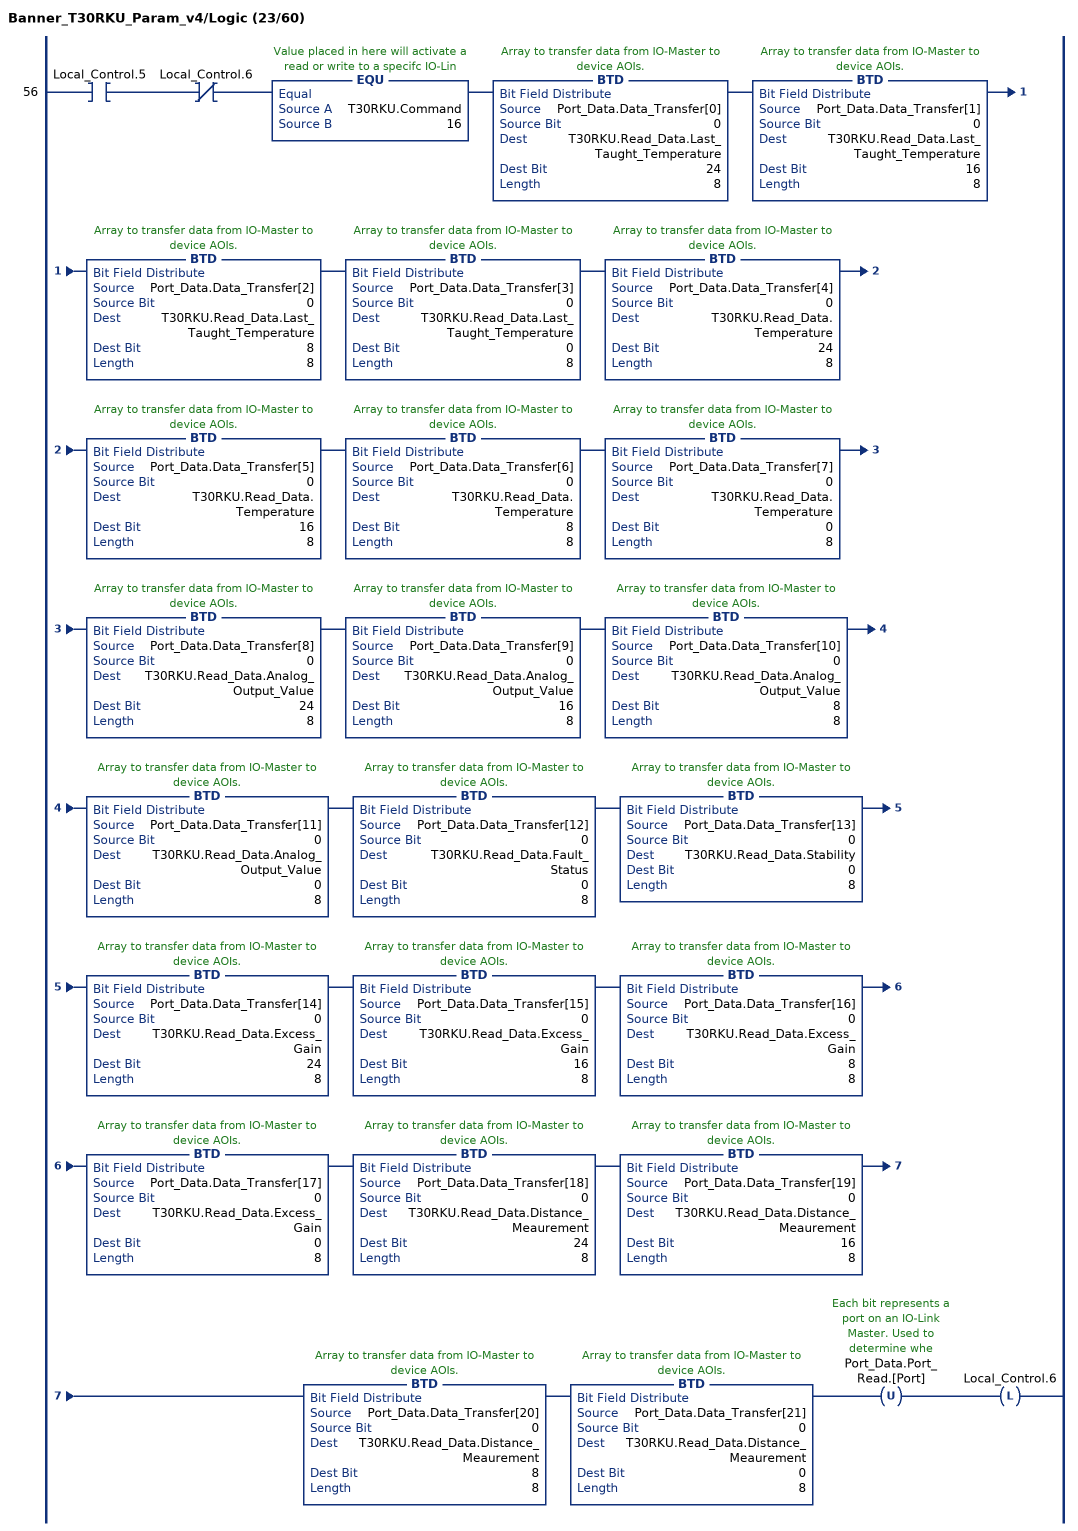
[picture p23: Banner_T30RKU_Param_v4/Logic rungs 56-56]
   56: XIC(Local_Control.5)XIO(Local_Control.6)EQU(T30RKU.Command,16)BTD(Port_Data.Data_Transfer[0],0,T30RKU.Read_Data.Last_Taught_Temperature,24,8)BTD(Port_Data.Data_Transfer[1],0,T30RKU.Read_Data.Last_Taught_Temperature,16,8)BTD(Port_Data.Data_Transfer[2],0,T30RKU.Read_Data.Last_Taught_Temperature,8,8)BTD(Port_Data.Data_Transfer[3],0,T30RKU.Read_Data.Last_Taught_Temperature,0,8)BTD(Port_Data.Data_Transfer[4],0,T30RKU.Read_Data.Temperature,24,8)BTD(Port_Data.Data_Transfer[5],0,T30RKU.Read_Data.Temperature,16,8)BTD(Port_Data.Data_Transfer[6],0,T30RKU.Read_Data.Temperature,8,8)BTD(Port_Data.Data_Transfer[7],0,T30RKU.Read_Data.Temperature,0,8)BTD(Port_Data.Data_Transfer[8],0,T30RKU.Read_Data.Analog_Output_Value,24,8)BTD(Port_Data.Data_Transfer[9],0,T30RKU.Read_Data.Analog_Output_Value,16,8)BTD(Port_Data.Data_Transfer[10],0,T30RKU.Read_Data.Analog_Output_Value,8,8)BTD(Port_Data.Data_Transfer[11],0,T30RKU.Read_Data.Analog_Output_Value,0,8)BTD(Port_Data.Data_Transfer[12],0,T30RKU.Read_Data.Fault_Status,0,8)BTD(Port_Data.Data_Transfer[13],0,T30RKU.Read_Data.Stability,0,8)BTD(Port_Data.Data_Transfer[14],0,T30RKU.Read_Data.Excess_Gain,24,8)BTD(Port_Data.Data_Transfer[15],0,T30RKU.Read_Data.Excess_Gain,16,8)BTD(Port_Data.Data_Transfer[16],0,T30RKU.Read_Data.Excess_Gain,8,8)BTD(Port_Data.Data_Transfer[17],0,T30RKU.Read_Data.Excess_Gain,0,8)BTD(Port_Data.Data_Transfer[18],0,T30RKU.Read_Data.Distance_Meaurement,24,8)BTD(Port_Data.Data_Transfer[19],0,T30RKU.Read_Data.Distance_Meaurement,16,8)BTD(Port_Data.Data_Transfer[20],0,T30RKU.Read_Data.Distance_Meaurement,8,8)BTD(Port_Data.Data_Transfer[21],0,T30RKU.Read_Data.Distance_Meaurement,0,8)OTU(Port_Data.Port_Read.[Port])OTL(Local_Control.6);
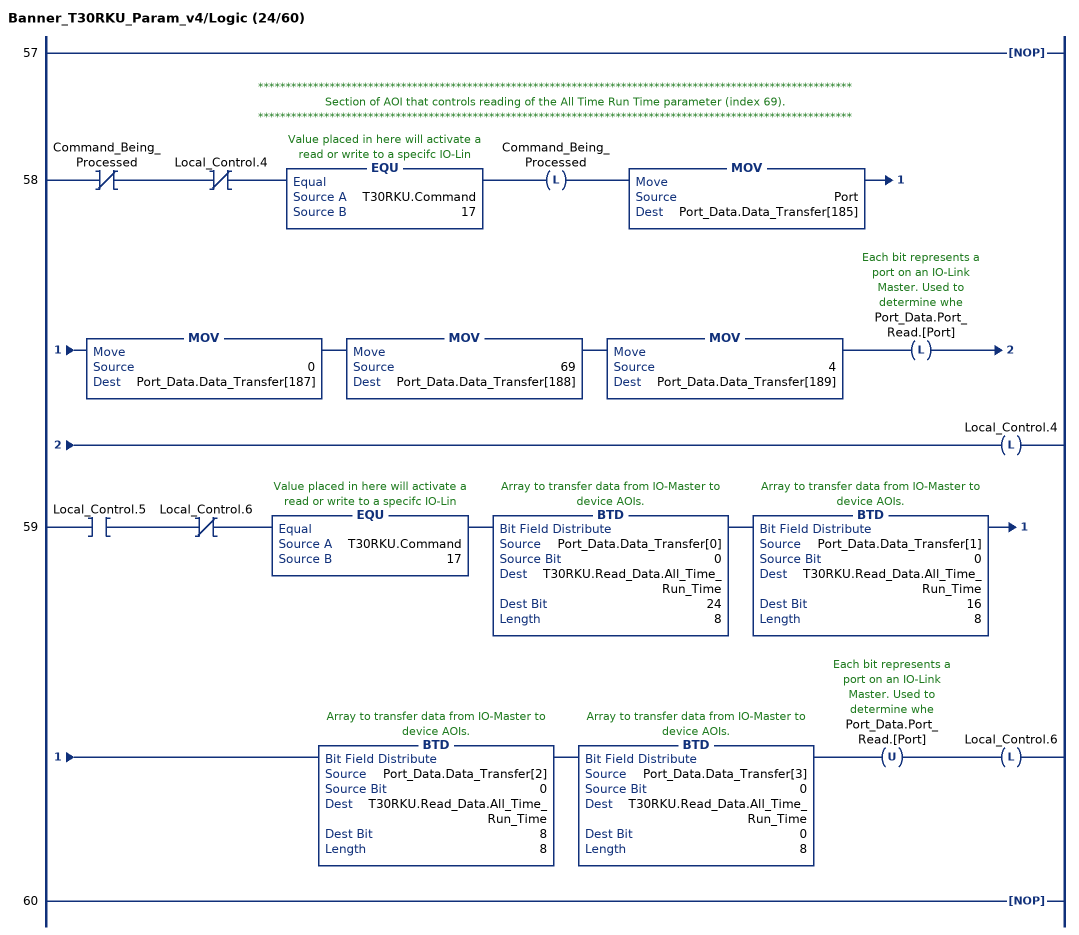
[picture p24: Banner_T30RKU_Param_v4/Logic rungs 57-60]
   57: NOP();
   // ************************************************************************************************************
   // Section of AOI that controls reading of the All Time Run Time parameter (index 69).
   // ************************************************************************************************************
   58: XIO(Command_Being_Processed)XIO(Local_Control.4)EQU(T30RKU.Command,17)OTL(Command_Being_Processed)MOV(Port,Port_Data.Data_Transfer[185])MOV(0,Port_Data.Data_Transfer[187])MOV(69,Port_Data.Data_Transfer[188])MOV(4,Port_Data.Data_Transfer[189])OTL(Port_Data.Port_Read.[Port])OTL(Local_Control.4);
   59: XIC(Local_Control.5)XIO(Local_Control.6)EQU(T30RKU.Command,17)BTD(Port_Data.Data_Transfer[0],0,T30RKU.Read_Data.All_Time_Run_Time,24,8)BTD(Port_Data.Data_Transfer[1],0,T30RKU.Read_Data.All_Time_Run_Time,16,8)BTD(Port_Data.Data_Transfer[2],0,T30RKU.Read_Data.All_Time_Run_Time,8,8)BTD(Port_Data.Data_Transfer[3],0,T30RKU.Read_Data.All_Time_Run_Time,0,8)OTU(Port_Data.Port_Read.[Port])OTL(Local_Control.6);
   60: NOP();
